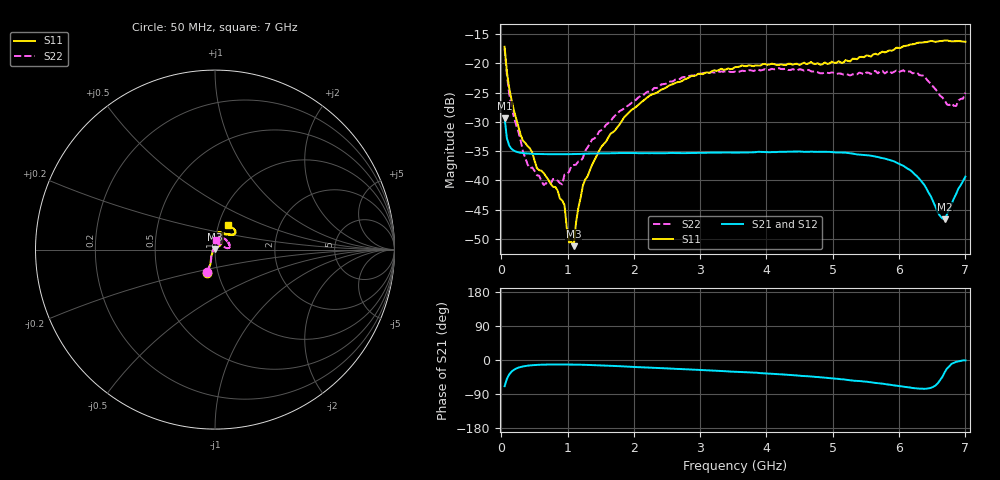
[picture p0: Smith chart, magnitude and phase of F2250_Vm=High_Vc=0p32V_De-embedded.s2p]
! Integrated Device Technology
! Corporate Headquarters
! 6024 Silver Creek Valley Road
! San Jose, CA 95138  USA
! Phone:  1-408-284-8200
! Toll Free:  1-800-223-1366
! Webpage:  http://www.idt.com/
! Timing and RF Division
! 515 Groton Road, Suite 102
! Westford, MA 01886-6024
! Device:  F2250
! Description: Voltage Variable RF Attenuator
! Frequency:  50.0 -  6000.00 MHz
! Package:  3x3 mm Thin QFN Plastic Package: 16 pin
! Ports:  2 RF, 3 DC
!  Pin  1  = GND
!  Pin  2  = NC
!  Pin  3  = RF1  = Port 1
!  Pin  4  = NC
!  Pin  5  = GND
!  Pin  6  = GND
!  Pin  7  = GND
!  Pin  8  = GND
!  Pin  9  = NC
!  Pin 10  = RF2  = Port 2
!  Pin 11  = NC
!  Pin 12  = GND
!  Pin 13  = GND
!  Pin 14  = VCNTRL
!  Pin 15  = VDD
!  Pin 16  = VMODE
! Vcntrl:  0.320 Volts
! Vmode:  +3.300 Volts
! Vdd:  +3.30  Volts
! Current:  1.257 mA
! Data:  The device was measured on a the F2250 evaluation board which has
!  individual transmission lines to the RF pins.  Data was collected
!  using a calibrated network analyzer.  The evaluation board was
!  de-embedded using a TRL calibration technique.
!  The reference plane is the edge of the package pin.
! Misc:  SN 10
!  Action Tracker AT0258
! Date Measured:  2014-11-26
! Date:  2015-10-15  MJV
! Note:
!  Integrated Device Technology supplies this data as a sample of measured
!  data at the package pin for this product.  Your particular data for this
!  product may vary.
!  Data was taken at 25 degrees C.
!  Integrated Device Technology reserves the right to change this data at anytime.
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# GHz S dB R 50
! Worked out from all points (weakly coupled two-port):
!   201 points, 50 MHz to 7 GHz, reference 50 ohm
!   highest |S21| = -29.35 dB at 50 MHz (marker M1); lowest = -46.6 dB at 6.687 GHz (marker M2)
!   lowest |S11| = -51.2 dB at 1.093 GHz (marker M3), VSWR 1.01, Z = 50 + j0.275 ohm
!   |S11| at or under -10 dB: start of sweep to end of sweep
!   |S22| runs from -40.8 to -17.5 dB; largest |S21 - S12| = 6.3e-05
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0.05  -17.18 -108.5  -29.35 -69.2  -29.36 -69.2  -17.47 -110.1
0.08475  -21.47 -107.4  -32.81 -49.8  -32.80 -49.8  -22.02 -107.8
0.189  -28.00 -120.0  -34.91 -26.0  -34.91 -26.0  -29.14 -121.6
0.29325  -32.26 -127.4  -35.28 -18.4  -35.27 -18.4  -33.26 -129.3
0.3975  -34.14 -142.2  -35.40 -15.0  -35.40 -15.0  -37.29 -154.7
0.5365  -37.89 -154.6  -35.47 -12.9  -35.47 -12.9  -39.10 -178.5
0.64075  -38.75 -162.6  -35.50 -12.2  -35.50 -12.2  -40.77 158.1
0.91875  -43.42 156.0  -35.52 -11.8  -35.52 -11.8  -40.67 119.2
0.9535  -44.22 170.9  -35.52 -11.8  -35.52 -11.8  -39.02 116.8
1.023  -50.58 140.3  -35.51 -11.9  -35.51 -11.9  -38.50 99.1
1.0925  -51.22 90.2  -35.50 -12.1  -35.50 -12.1  -37.37 90.0
1.12725  -47.19 61.6  -35.49 -12.2  -35.48 -12.2  -37.30 82.9
1.2315  -40.84 40.6  -35.44 -12.6  -35.44 -12.6  -36.13 69.1
1.6485  -32.01 41.2  -35.36 -15.3  -35.36 -15.3  -29.88 56.0
2.37825  -24.76 46.7  -35.32 -21.2  -35.33 -21.2  -24.05 51.9
3.525  -20.65 71.7  -35.25 -30.8  -35.25 -30.9  -21.42 71.9
4.7065  -20.06 72.0  -35.10 -44.1  -35.09 -44.2  -21.41 69.7
5.85325  -17.79 40.5  -36.50 -65.0  -36.51 -65.2  -21.27 22.4
6.3745  -16.40 40.9  -40.66 -76.0  -40.69 -76.1  -22.09 6.2
6.68725  -16.11 47.8  -46.64 -32.6  -46.63 -32.2  -26.30 27.6
6.861  -16.22 54.5  -42.29 -4.9  -42.25 -4.9  -27.28 57.6
7  -16.32 62.4  -39.35 -1.0  -39.31 -1.2  -25.02 84.4
